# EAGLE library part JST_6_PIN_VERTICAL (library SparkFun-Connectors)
JST 6 pin vertical connector Here is a six pin vertical 1.0mm pitch connector. It is useful if you need something very tiny as a connection. These are not the standard JST type connectors we use on most of our boards, but are actually the much smaller JST-SH type. Here is the connector we sell at SparkFun: JST SH Vertical 6-Pin Connector - SMD (GPS-00579) Datasheet It was used on these SparkFun products: SparkFun GPS Breakout (BOB-11818) SparkFun Weather Shield (DEV-12081) And many, many other GPS related products.
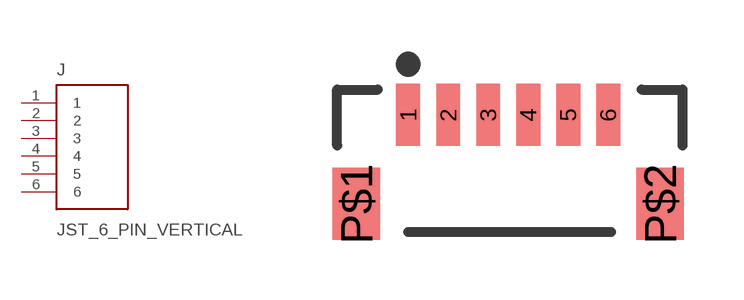
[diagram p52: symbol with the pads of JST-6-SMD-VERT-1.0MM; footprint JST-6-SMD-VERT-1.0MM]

Designator prefix J

## JST_6_PIN_VERTICAL (PROD_ID: CONN-08249; SF_ID: GPS-00579)  [JST-6-SMD-VERT-1.0MM]
1  1
2  2
3  3
4  4
5  5
6  6

## Footprint JST-6-SMD-VERT-1.0MM (pad centres in mm)
JST SH Vertical 6-Pin SMT Specifications: Pin count:6 Pin pitch: 1 mm Datasheet referenced for footprint Example device(s): JST_6PIN_VERTICAL
smd 0.6 x 1.55: 1 -2.54,1.27; 2 -1.54,1.27; 3 -0.54,1.27; 4 0.46,1.27; 5 1.46,1.27; 6 2.46,1.27
smd 1.2 x 1.8: P$1 -3.84,-0.955; P$2 3.76,-0.955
